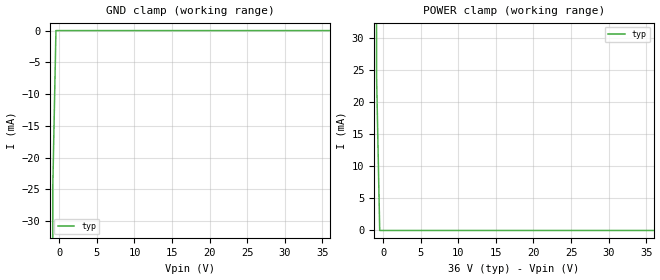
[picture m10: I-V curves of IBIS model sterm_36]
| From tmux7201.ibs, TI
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| sterm_36
[Model]   sterm_36
Model_type   Terminator
|   typ   min   max
C_comp   4.014581e-11   NA   NA
[Voltage Range]   36   NA   NA
[Temperature Range]   27   NA   NA
[Power Clamp Reference]   36   NA   NA
[GND Clamp Reference]   0   NA   NA
[GND Clamp]
|   Voltage   I(typ)   I(min)   I(max)
-5V       -10.46A    NA         NA
-1.273V   -621.4mA   NA         NA
-858.6mV  -24.21mA   NA         NA
-444.4mV  -30.96nA   NA         NA
36V       1.41nA     NA         NA
[POWER Clamp]
|   Voltage   I(typ)   I(min)   I(max)
-5V       13.27A     NA         NA
-1.273V   611.4mA    NA         NA
-858.6mV  23.93mA    NA         NA
-444.4mV  23.28nA    NA         NA
36V       -1.411nA   NA         NA
